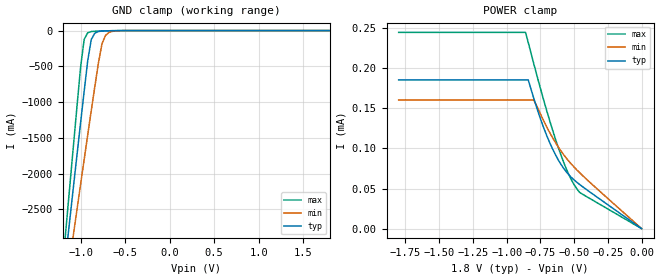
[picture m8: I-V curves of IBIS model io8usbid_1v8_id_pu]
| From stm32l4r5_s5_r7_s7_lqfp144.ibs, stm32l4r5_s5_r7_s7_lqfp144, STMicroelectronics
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|   Model io8usbid_1v8_id_pu
[Model]  io8usbid_1v8_id_pu
Model_type Input
Polarity   Non-Inverting
Vinl =   0.540000V
Vinh =   1.260000V
C_comp   2.031500pF   1.968500pF   2.084900pF
[Temperature Range]   25.000000   0.125000k   -40.000000
[Pullup Reference]   1.800000V   1.600000V   2.000000V
[Pulldown Reference]   0.0V   0.0V   0.0V
[POWER Clamp Reference]   1.800000V   1.600000V   2.000000V
[GND Clamp Reference]   0.0V   0.0V   0.0V
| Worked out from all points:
|   GND clamp passes 1 mA (typ) near -0.60 V on its own axis
[GND_clamp]
|Voltage   I(typ)   I(min)   I(max)
-1.8V     -9.895A    -9.296A    -9.457A
-1.2V     -3.533A    -3.902A    -3.274A
-1.16V    -3.082A    -3.55A     -2.716A
-1.12V    -2.631A    -3.198A    -2.159A
-1.08V    -2.182A    -2.848A    -1.604A
-1V       -1.289A    -2.15A     -512mA
-960mV    -849.4mA   -1.803A    -123.8mA
-920mV    -422.4mA   -1.459A    -30.79mA
-880mV    -123.7mA   -1.118A    -13.63mA
-760mV    -6.32mA    -185mA     -5.692mA
-680mV    -2.569mA   -25.43mA   -2.907mA
1.8V      0A         0A         0A
[POWER_clamp]
|Voltage   I(typ)   I(min)   I(max)
-1.8V     185.5uA    160.5uA    244.8uA
-860mV    185.5uA    160.5uA    244.8uA
-840mV    185.5uA    160.5uA    232.3uA
-800mV    163.2uA    160.5uA    206.4uA
-720mV    123.4uA    132.6uA    157.1uA
-660mV    99.54uA    113.5uA    123.2uA
-620mV    86.5uA     102.5uA    102.5uA
-580mV    75.76uA    92.77uA    83.86uA
-540mV    67.29uA    84.27uA    67.7uA
-500mV    60.7uA     76.74uA    54.84uA
-460mV    55.2uA     69.91uA    45.31uA
0V        0A         0A         0A
